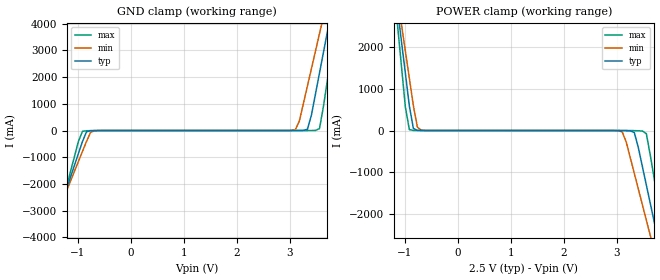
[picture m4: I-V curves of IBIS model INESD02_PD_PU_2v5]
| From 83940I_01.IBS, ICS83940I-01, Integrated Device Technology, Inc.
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[Model] INESD02_PD_PU_2v5
Model_type   Input
Polarity   Non-Inverting
Vinl = 0.8V
Vinh = 2.0V
|   typ   min   max
C_comp   2pF   1.5pF   2.5pF
|   typ   min   max
[Voltage range]  2.5V   2.375V   2.625V
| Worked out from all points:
|   GND clamp passes 1 mA (typ) near -0.59 V on its own axis
|   POWER clamp passes 1 mA (typ) near -0.69 V on its own axis
[GND_clamp]
|Voltage I(typ)   I(min)   I(max)
-2.5V     -9.8A      -8.606A    -11.82A
-1.591V   -4.431A    -4.131A    -4.968A
-1.439V   -3.536A    -3.386A    -3.826A
-909.1mV  -407.2mA   -779mA     -28.28mA
-833.3mV  -48.54mA   -407.3mA   -8.383mA
-681.8mV  -2.93mA    -9.176mA   -2.087mA
3.106V    184.5uA    34.21mA    58.45uA
3.333V    47.83mA    1.665A     150.4uA
3.561V    2.15A      3.624A     71.91mA
3.712V    3.718A     4.931A     1.914A
3.864V    5.287A     6.238A     3.919A
5V        17.07A     16.05A     18.97A
[POWER_clamp]
|Voltage   I(typ)   I(min)   I(max)
-2.5V     17.07A     14.97A     20.63A
-1.136V   2.934A     3.199A     2.565A
-1.061V   2.15A      2.546A     1.563A
-909.1mV  582.5mA    1.24A      20.76mA
-833.3mV  47.83mA    588.2mA    1.398mA
-681.8mV  605.5uA    7.845mA    110.4uA
3.106V    -1.193mA   -33.42mA   -88.57uA
3.333V    -48.54mA   -1.021A    -2.868mA
3.485V    -853.7mA   -1.765A    -10.73mA
3.712V    -2.194A    -2.883A    -1.171A
3.939V    -3.536A    -4.001A    -2.884A
5V        -9.8A      -9.222A    -10.88A
